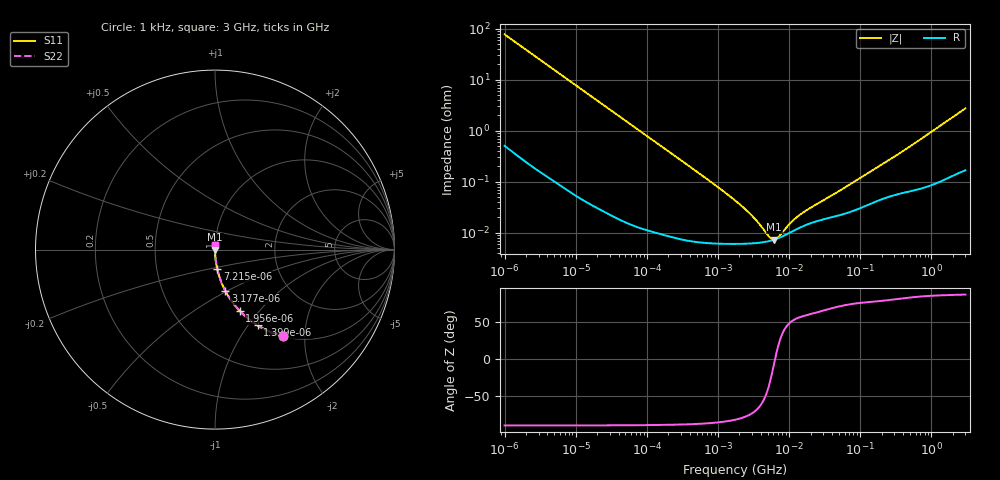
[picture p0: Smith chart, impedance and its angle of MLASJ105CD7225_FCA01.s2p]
! MLASJ105CD7225_FCA01  S-PARAMETER MODEL  ( Standard Model )
! Model Generated by TAIYO YUDEN Corporation (http://www.ty-top.com)
! Version 1.0
! TAIYO YUDEN Control No. 240524
! Copyright(c) 2024 TAIYO YUDEN CO.,LTD. All Rights Reserved.
! Product Description (link to TY-COMPAS)
! https://ds.yuden.co.jp/TYCOMPAS/or/detail?pn=MLASJ105CD7225KFCA01&u=M
! Products Name : Multilayer Ceramic Capacitors
! Characteristics :
!  Capacitance : 2.2 [uF] , Rated Voltage : 6.3 [V] , TCC : X7T
!  Case Size : 1.0 x 0.5 / 0.039 x 0.02 [mm/inch] , Thickness : 0.5 / 0.02 [mm/inch]
!  (Conditions: Temperature = 25 [degC] , DC Bias Voltage = 0 [V])
! External Node Assignments :
!  1  o---| |---o  2
! GND o---------o GND
! Frequency Range : 1kHz  -  3GHz  [ 401 STEP ]
# MHZ S RI R 50
! Freq[MHz].  S11 Real  S11 Imag  S21 Real  S21 Imag  S12 Real  S12 Imag  S22 Real  S22 Imag
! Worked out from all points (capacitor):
!   401 points, 1 kHz to 3 GHz, reference 50 ohm
!   read as one part in series: C = 2.05 uF near 1.077 kHz
!   lowest |Z| = 7.32 mohm at 6.153 MHz (marker M1)
!   series resonance near 6.348 MHz, so ESL is about 310 pH
!   S11 on the Smith chart (normalised r, x): 1 kHz: 1.01, -1.55; 1.399 kHz: 1.01, -1.11; 1.956 kHz: 1.00, -0.80; 3.177 kHz: 1.00, -0.49; 7.215 kHz: 1.00, -0.22; 3 GHz: 1.00, +0.05
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0.001  0.3764 -0.4812  0.6236 0.4812  0.6236 0.4812  0.3764 -0.4812
0.001399  0.2371 -0.4221  0.7629 0.4221  0.7629 0.4221  0.2371 -0.4221
0.001956  0.138 -0.3418  0.862 0.3418  0.862 0.3418  0.138 -0.3418
0.003177  0.058 -0.2307  0.942 0.2307  0.942 0.2307  0.058 -0.2307
0.004787  0.0268 -0.1584  0.9732 0.1584  0.9732 0.1584  0.0268 -0.1584
0.007215  0.0123 -0.1069  0.9877 0.1069  0.9877 0.1069  0.0123 -0.1069
0.01216  0.00457 -0.0641  0.9954 0.0641  0.9954 0.0641  0.00457 -0.0641
0.033275  0.000766 -0.0236  0.9992 0.0236  0.9992 0.0236  0.000766 -0.0236
0.147855  0.000124 -0.00535  0.9999 0.00535  0.9999 0.00535  0.000124 -0.00535
0.762639  6.28e-05 -0.00103  0.9999 0.00103  0.9999 0.00103  6.28e-05 -0.00103
1.732051  6.02e-05 -0.000426  0.9999 0.000426  0.9999 0.000426  6.02e-05 -0.000426
2.919173  6.13e-05 -0.000215  0.9999 0.000215  0.9999 0.000215  6.13e-05 -0.000215
4.566395  6.57e-05 -8.35e-05  0.9999 8.35e-05  0.9999 8.35e-05  6.57e-05 -8.35e-05
5.106836  6.78e-05 -5.44e-05  0.9999 5.44e-05  0.9999 5.44e-05  6.78e-05 -5.44e-05
6.153411  7.28e-05 -7.61e-06  0.9999 7.61e-06  0.9999 7.61e-06  7.28e-05 -7.61e-06
7.414467  8.02e-05 3.76e-05  0.9999 -3.76e-05  0.9999 -3.76e-05  8.02e-05 3.76e-05
7.988506  8.39e-05 5.53e-05  0.9999 -5.53e-05  0.9999 -5.53e-05  8.39e-05 5.53e-05
12.49624  0.000115 0.000158  0.9999 -0.000158  0.9999 -0.000158  0.000115 0.000158
21.06097  0.000157 0.000281  0.9998 -0.000281  0.9998 -0.000281  0.000157 0.000281
49.64928  0.000217 0.000608  0.9998 -0.000608  0.9998 -0.000608  0.000217 0.000608
256.0921  0.000515 0.00264  0.9995 -0.00264  0.9995 -0.00264  0.000515 0.00264
3000  0.00241 0.0272  0.9976 -0.0272  0.9976 -0.0272  0.00241 0.0272
